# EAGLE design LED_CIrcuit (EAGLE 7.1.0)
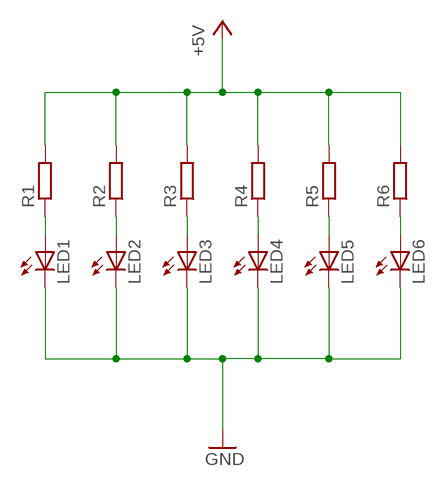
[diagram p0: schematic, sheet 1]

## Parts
LED1  LEDCHIPLED_0603  [CHIPLED_0603]
LED2  LEDCHIPLED_0603  [CHIPLED_0603]
LED3  LEDCHIPLED_0603  [CHIPLED_0603]
LED4  LEDCHIPLED_0603  [CHIPLED_0603]
LED5  LEDCHIPLED_0603  [CHIPLED_0603]
LED6  LEDCHIPLED_0603  [CHIPLED_0603]
R1  R-EU_R0603  [R0603]
R2  R-EU_R0603  [R0603]
R3  R-EU_R0603  [R0603]
R4  R-EU_R0603  [R0603]
R5  R-EU_R0603  [R0603]
R6  R-EU_R0603  [R0603]

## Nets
+5V: R1.2 R2.2 R3.2 R4.2 R5.2 R6.2
GND: LED1.C LED2.C LED3.C LED4.C LED5.C LED6.C
N$1: LED1.A R1.1
N$3: LED2.A R2.1
N$4: LED3.A R3.1
N$5: LED4.A R4.1
N$6: LED5.A R5.1
N$7: LED6.A R6.1

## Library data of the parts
LED1-LED6 = led:LED: LED
R1-R6 = rcl:R-EU_: RESISTOR, European symbol

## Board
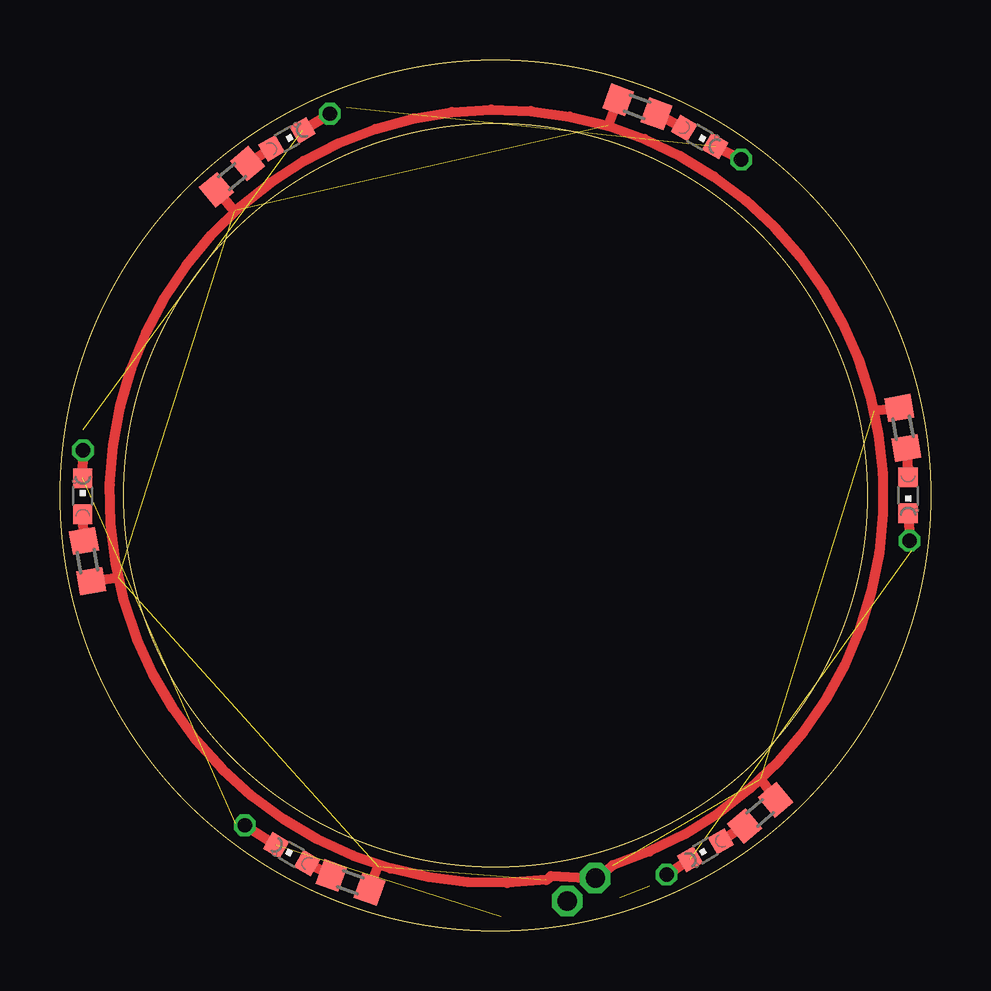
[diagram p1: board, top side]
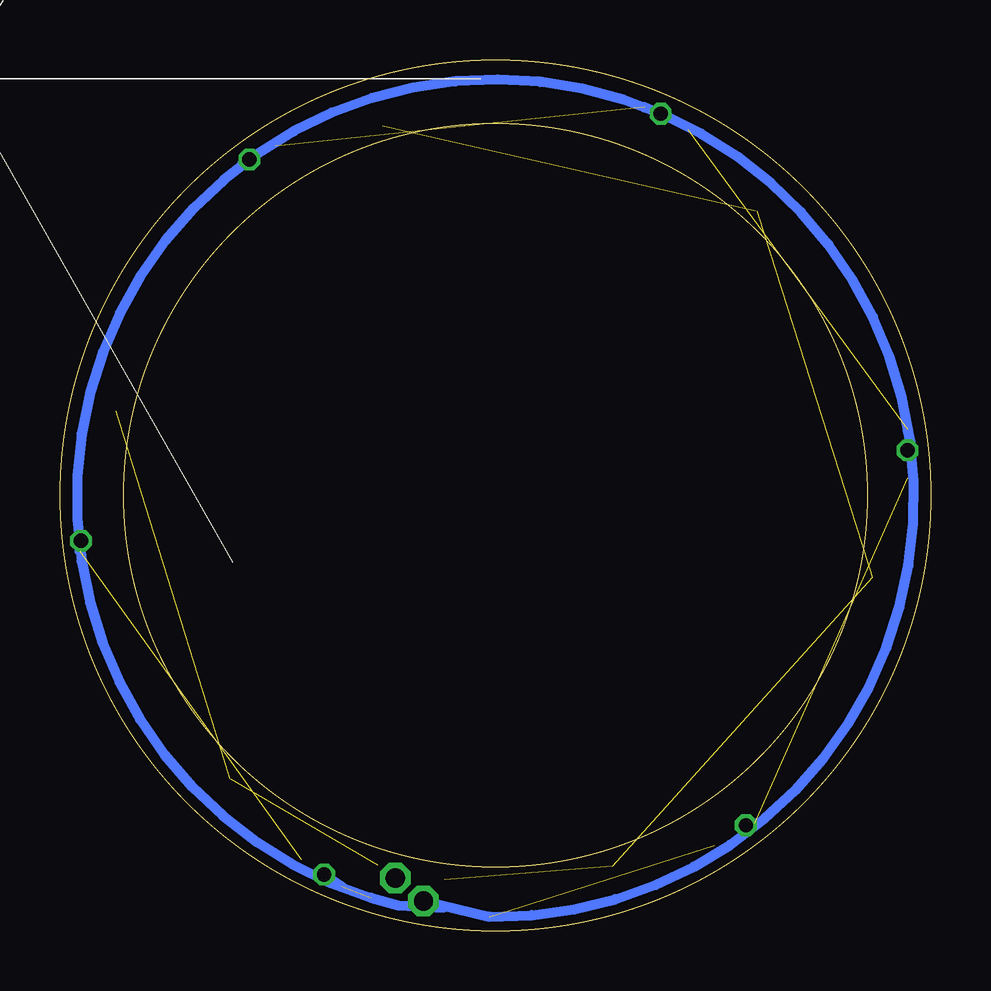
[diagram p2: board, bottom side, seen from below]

Size 36.3 x 36.3 mm. Coordinates in mm from the lower left corner, seen from the top.
Outline: circle at 18.15,18.15 radius 18.15
Outline: circle at 18.15,18.15 radius 15.5
Copper layers (1*16): Top 0.035mm / dielectric 1.5mm / Bottom 0.035mm
Design rules "PCB-POOL Standard": minimum track width 0.15mm, minimum drill 0.3mm, track to track 0.15mm, track to pad 0.15mm, pad to pad 0.15mm, via to via 0.15mm, smd to smd 0.15mm, copper to edge 0.3mm, drill to drill 0.2mm, minimum pad ring 0.2mm, minimum via ring 0.15mm, stop-mask expansion 0.075mm, vias tented up to drill 0mil, thermal gap 0.2mm

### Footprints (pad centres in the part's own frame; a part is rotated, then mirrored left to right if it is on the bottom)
CHIPLED_0603 = smd 0.8 x 0.8: A 0,-0.75; C 0,0.75
R0603 = smd 1 x 1.1: 1 -0.85,0; 2 0.85,0

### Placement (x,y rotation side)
LED1  9.66,3.19 60 top
LED2  0.95,18.12 0 top
LED3  9.46,32.99 300 top
LED4  26.67,33.09 240 top
LED5  35.36,18.15 180 top
LED6  26.91,3.35 120 top
R1  12.11,2.02 340 top
R2  1.15,15.41 280 top
R3  7.17,31.44 220 top
R4  24.07,34.34 160 top
R5  35.14,20.96 100 top
R6  29.19,4.91 40 top

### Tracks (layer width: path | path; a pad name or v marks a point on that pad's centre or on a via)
+5V  (via drill 0.8 pad 1.27)  (6 unrouted)
  Top 0.406: R1.2 13.26,2.69 | R2.2 2.44,14.73 | R3.2 7.26,30.01 7.26,30.02 7.3,30.03 | R5.2 33.95,21.67 | R6.2 29.22,6.33 29.17,6.32 29.26,6.31 | R4.2 22.85,33.55 | v22.32,2.19 23.05,2.73 arc350 20.27,2.12 20.39,2.2 20.46,2.28 v22.32,2.19
GND  (via drill 0.6, 0.8 pad 1.27)  (6 unrouted)
  Top 0.406: LED1.C v7.71,4.4 | LED2.C v0.96,20.02 | LED3.C v11.25,34.06 | LED4.C v28.4,32.15 | LED5.C v35.42,16.26 | LED6.C v25.29,2.34
  Bottom 0.406: v7.71,4.4 7.33,4.47 | v0.96,20.02 0.84,20.36 0.96,20.89 | v11.25,34.06 11.49,34.14 11.94,34.32 11.94,34.34 | v28.4,32.15 28.71,31.98 | v35.42,16.26 35.48,15.82 | v25.29,2.34 24.57,1.85 | v21.15,1.24 18.4,0.58 arc-344 23.34,1.37 22.2,1.06 20.29,0.96
N$1
  Top 0.406: R1.1 LED1.A
N$3
  Top 0.406: R2.1 LED2.A
N$4
  Top 0.406: R3.1 LED3.A
N$5
  Top 0.406: R4.1 LED4.A
N$6
  Top 0.406: R5.1 LED5.A
N$7
  Top 0.406: LED6.A R6.1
